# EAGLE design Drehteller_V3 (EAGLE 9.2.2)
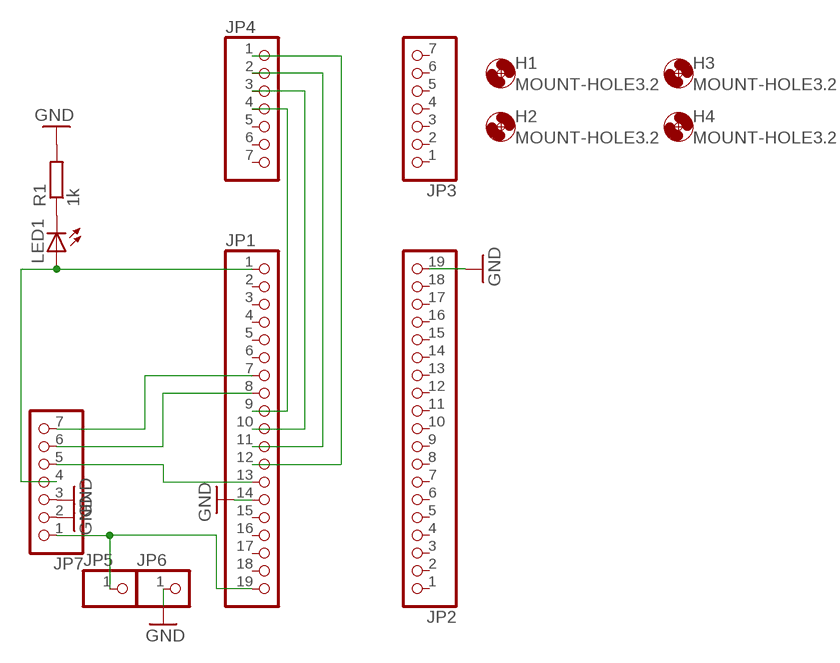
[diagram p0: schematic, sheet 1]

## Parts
H1  MOUNT-HOLE3.2  [3,2]
H2  MOUNT-HOLE3.2  [3,2]
H3  MOUNT-HOLE3.2  [3,2]
H4  MOUNT-HOLE3.2  [3,2]
JP1  PINHD-1X19  [1X19]
JP2  PINHD-1X19  [1X19]
JP3  PINHD-1X7  [1X07]
JP4  PINHD-1X7  [1X07]
JP5  PINHD-1X1  [1X01]
JP6  PINHD-1X1  [1X01]
JP7  PINHD-1X7  [1X07]
LED1  LED5MM  [LED5MM]
R1  1k  R-EU_0207/10  [0207/10]

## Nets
GND: JP1.14 JP2.19 JP6.1 JP7.2 JP7.3 R1.2
N$1: JP1.12 JP4.1
N$2: JP1.11 JP4.2
N$3: JP1.10 JP4.3
N$4: JP1.9 JP4.4
N$5: JP1.19 JP5.1 JP7.1
N$6: JP1.7 JP7.7
N$7: JP1.1 JP7.4 LED1.A
N$8: LED1.K(C) R1.1
N$9: JP1.8 JP7.6
N$10: JP1.13 JP7.5
Unconnected: JP1.2 JP1.3 JP1.4 JP1.5 JP1.6 JP1.15 JP1.16 JP1.17 JP1.18 JP2.1 JP2.2 JP2.3 JP2.4 JP2.5 JP2.6 JP2.7 JP2.8 JP2.9 JP2.10 JP2.11 JP2.12 JP2.13 JP2.14 JP2.15 JP2.16 JP2.17 JP2.18 JP3.1 JP3.2 JP3.3 JP3.4 JP3.5 JP3.6 JP3.7 JP4.5 JP4.6 JP4.7

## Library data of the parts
H1-H4 = holes:MOUNT-HOLE: MOUNTING HOLE with drill center marker
JP1 JP2 = pinhead:PINHD-1X19: PIN HEADER
JP3 JP4 JP7 = pinhead:PINHD-1X7: PIN HEADER
JP5 JP6 = pinhead:PINHD-1X1: PIN HEADER
LED1 = led:LED: LED
R1 = rcl:R-EU_: RESISTOR, European symbol

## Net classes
0 default: clearance 0.205 mm

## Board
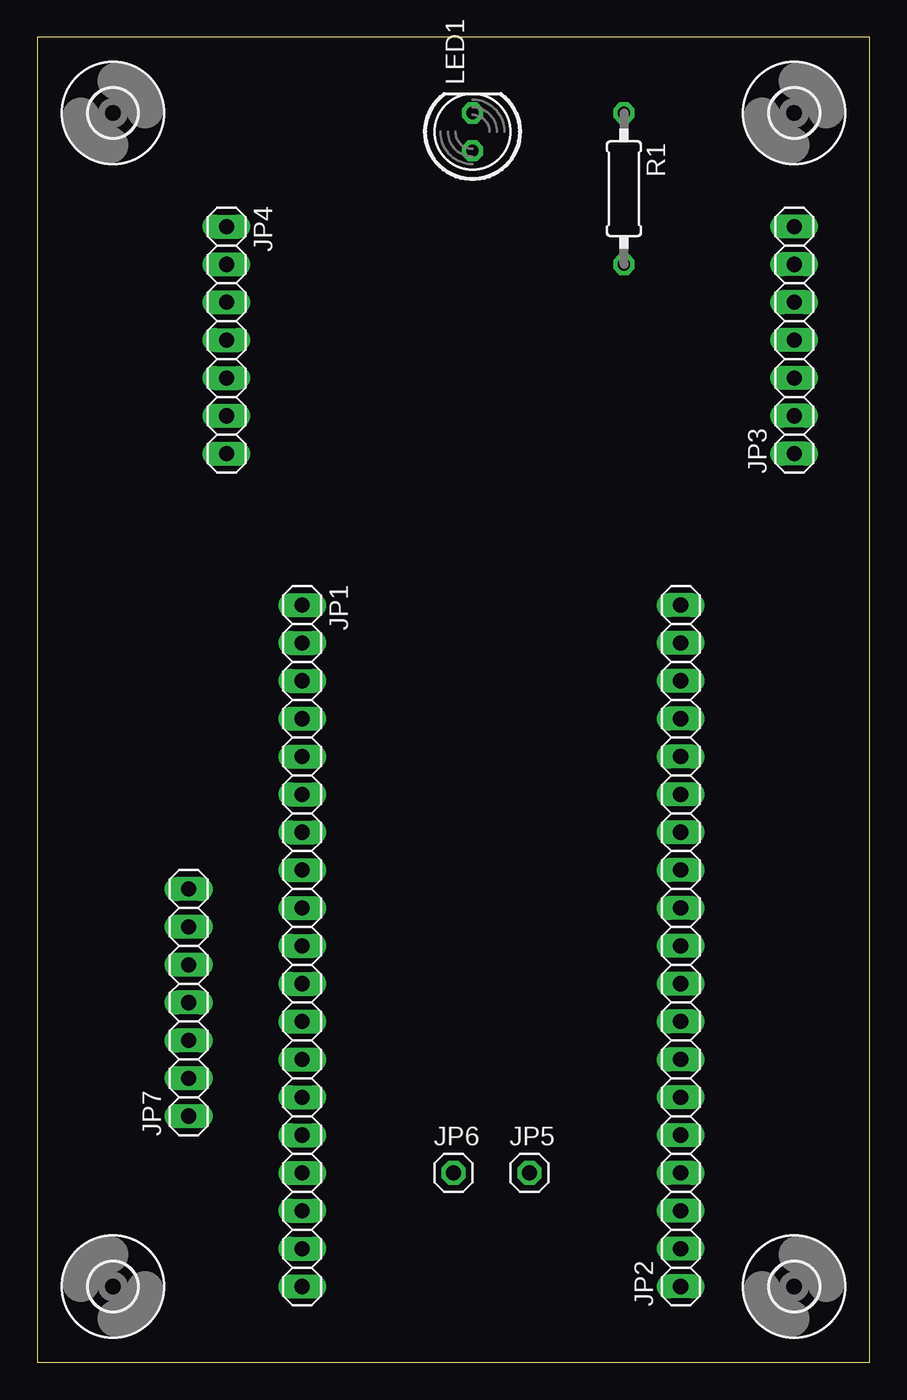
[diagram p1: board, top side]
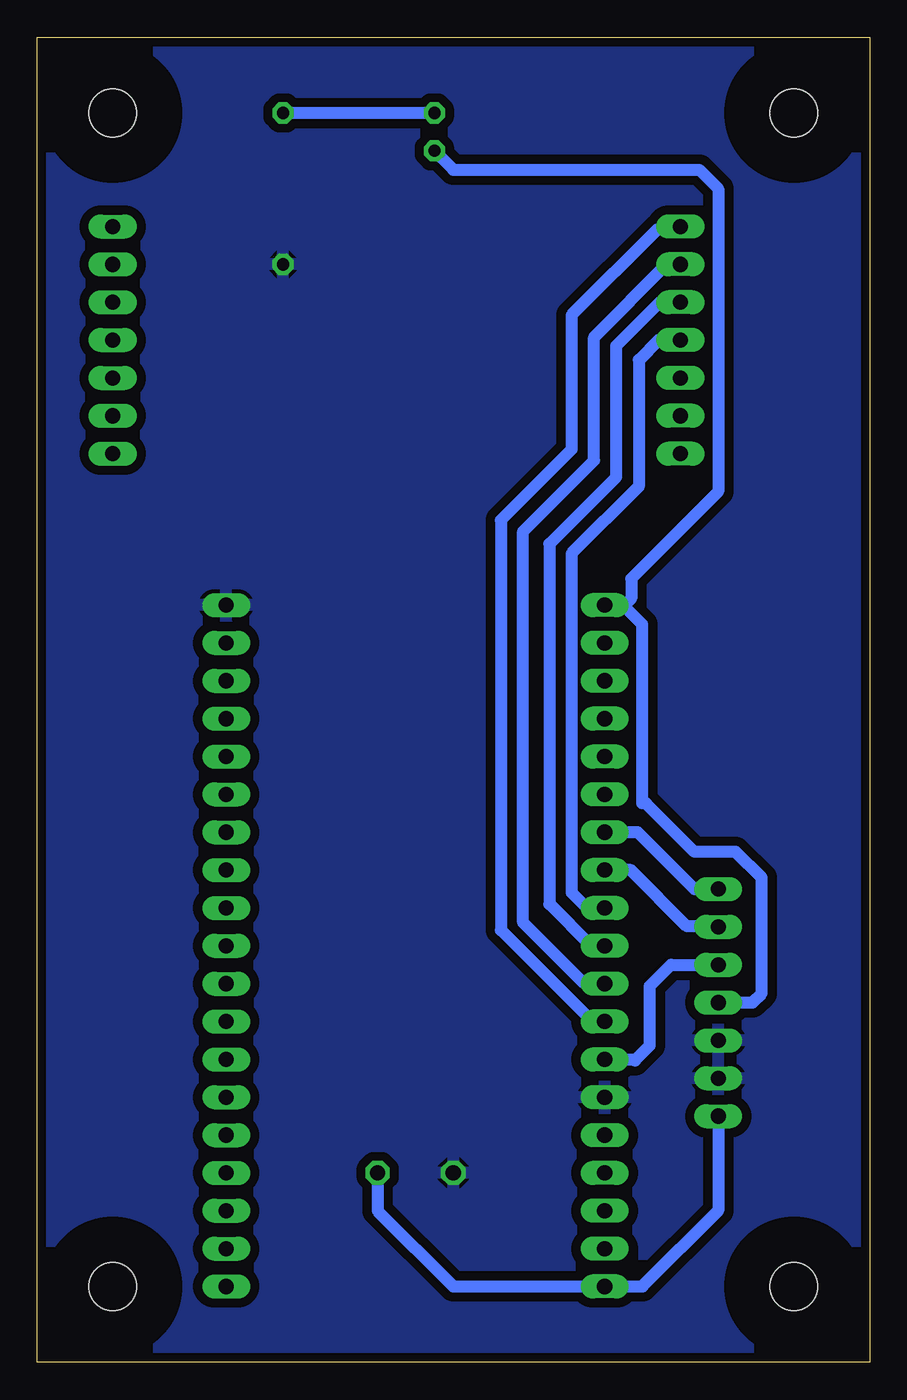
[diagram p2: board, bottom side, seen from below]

Size 55.86 x 88.9 mm. Coordinates in mm from the lower left corner, seen from the top.
Outline: 0,0 55.86,0 55.86,88.9 0,88.9 0,0
Copper layers (1*16): Top 0.035559375mm / dielectric 1.501140625mm / Bottom 0.035559375mm
Design rules "circuitcam": minimum track width 0.3mm, minimum drill 23mil, track to track 0.2mm, track to pad 0.2mm, pad to pad 0.2mm, via to via 0.2mm, smd to smd 0.2mm, copper to edge 0.5mm, drill to drill 8mil, minimum pad ring 0.3mm, minimum via ring 0.3mm, stop-mask expansion 4mil, vias tented up to drill 0mil, thermal gap 10mil

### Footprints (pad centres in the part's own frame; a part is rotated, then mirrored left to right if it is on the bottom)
3,2 = hole 3.2: 0,0
1X19 = drill 1.016 long: 1 -22.86,0; 2 -20.32,0; 3 -17.78,0; 4 -15.24,0; 5 -12.7,0; 6 -10.16,0; 7 -7.62,0; 8 -5.08,0; 9 -2.54,0; 10 0,0; 11 2.54,0; 12 5.08,0; 13 7.62,0; 14 10.16,0; 15 12.7,0; 16 15.24,0; 17 17.78,0; 18 20.32,0; 19 22.86,0
1X07 = drill 1.016 long: 1 -7.62,0; 2 -5.08,0; 3 -2.54,0; 4 0,0; 5 2.54,0; 6 5.08,0; 7 7.62,0
1X01 = drill 1.016 octagon: 1 0,0
LED5MM = drill 0.813 octagon: A -1.27,0; K 1.27,0
0207/10 = drill 0.813 octagon: 1 -5.08,0; 2 5.08,0

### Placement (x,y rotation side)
H1  50.8,5.08 0 top
H2  50.8,83.82 0 top
H3  5.08,83.82 180 top
H4  5.08,5.08 270 top
JP1  17.78,27.94 270 top
JP2  43.18,27.94 90 top
JP3  50.8,68.58 90 top
JP4  12.7,68.58 270 top
JP5  33.02,12.7 0 top
JP6  27.94,12.7 0 top
JP7  10.16,24.13 90 top
LED1  29.21,82.55 90 top
R1  39.37,78.74 270 top

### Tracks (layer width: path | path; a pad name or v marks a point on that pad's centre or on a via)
GND
  pour Bottom (isolate 0.61, rank 2): 0,88.9 0,0 55.88,0 55.88,88.9
N$1
  Bottom 0.813: JP4.1 12.9,76 14.25,76 20,70.25 20,61.25 24.75,56.5 24.75,29 18.61,22.86 JP1.12
N$2
  Bottom 0.813: JP1.11 17.88,25.5 19.25,25.5 23.25,29.5 23.25,55.75 18.5,60.5 18.5,68.75 13.59,73.66 JP4.2
N$3
  Bottom 0.813: JP4.3 14.08,71.12 17,68.2 17,59.4 21.5,54.9 21.5,30.75 18.69,27.94 JP1.10
N$4
  Bottom 0.813: JP4.4 14.17,68.58 15.5,67.25 15.5,58.75 20,54.25 20,51.4 20.01,51.39 20.01,31.51 19,30.5 18.75,30.5 18.73,30.48 JP1.9
N$5
  Bottom 0.813: JP7.1 10.16,10.16 15.24,5.08 JP1.19 27.94,5.08 33.02,10.16 JP5.1
N$6
  Bottom 0.813: JP7.7 11.75,31.75 15.56,35.56 JP1.7
N$7
  Bottom 0.813: LED1.A 27.94,80.01 11.43,80.01 10.16,78.74 10.16,58.42 16,52.58 16,51.25 16.45,50.8 JP1.1 17.54,51.04 16.79,51.04 15.25,49.5 15.25,37.5 15,37.5 11.75,34.25 9,34.25 7.25,32.5 7.25,24.75 7.87,24.13 JP7.4
N$8
  Bottom 0.813: LED1.K R1.1
N$9
  Bottom 0.813: JP7.6 10.2,29.25 12.25,29.25 16.02,33.02 JP1.8
N$10
  Bottom 0.813: JP1.13 15.82,20.32 15.75,20.25 14.75,21.25 14.75,25.25 13.33,26.67 JP7.5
